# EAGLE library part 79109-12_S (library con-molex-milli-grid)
RECEPTACAL
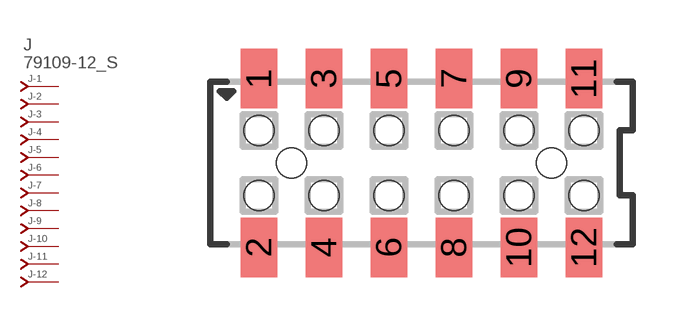
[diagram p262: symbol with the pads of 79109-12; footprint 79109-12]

Designator prefix J; gates -1=J-NV -2=J-N -3=J-N -4=J-N -5=J-N -6=J-N -7=J-N -8=J-N -9=J-N -10=J-N -11=J-N -12=J-N

## 79109-12_S  [79109-12]
1  -1:J  pas
2  -2:J  pas
3  -3:J  pas
4  -4:J  pas
5  -5:J  pas
6  -6:J  pas
7  -7:J  pas
8  -8:J  pas
9  -9:J  pas
10  -10:J  pas
11  -11:J  pas
12  -12:J  pas

## Footprint 79109-12 (pad centres in mm)
RECEPTACAL SMD Dual Row, Vertical, Pass-Thru
smd 1.12 x 1.83: 1 -5,2.6; 2 -5,-2.6; 3 -3,2.6; 4 -3,-2.6; 5 -1,2.6; 6 -1,-2.6; 7 1,2.6; 8 1,-2.6; 9 3,2.6; 10 3,-2.6; 11 5,2.6; 12 5,-2.6
hole 0.914 at -4,0
hole 0.914 at -5,1
hole 0.914 at -5,-1
hole 0.914 at -3,-1
hole 0.914 at -3,1
hole 0.914 at -1,-1
hole 0.914 at -1,1
hole 0.914 at 4,0
hole 0.914 at 1,1
hole 0.914 at 1,-1
hole 0.914 at 3,1
hole 0.914 at 3,-1
hole 0.914 at 5,1
hole 0.914 at 5,-1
